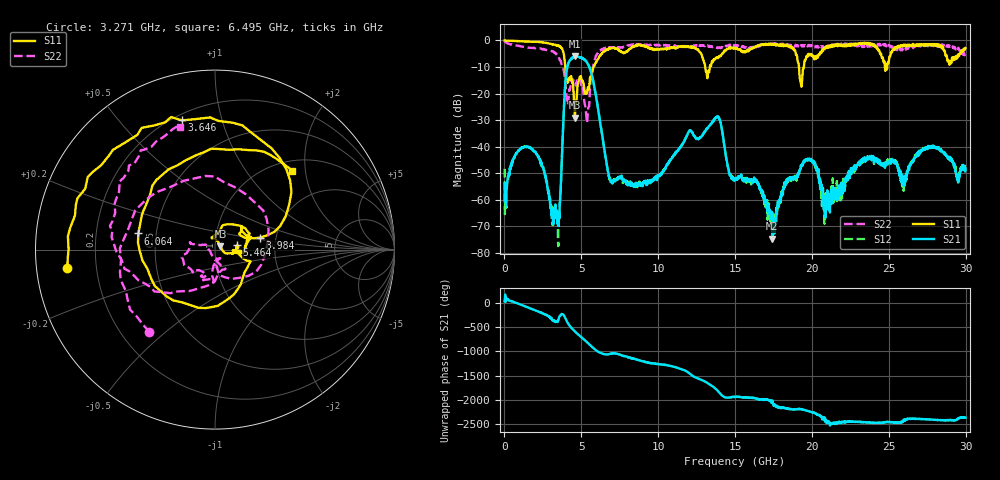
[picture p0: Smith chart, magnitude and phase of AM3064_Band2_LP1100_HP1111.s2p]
# Hz S DB R 50.0
!freq dBS11 angS11 dBS21 angS21 dBS12 angS12 dBS22 angS22
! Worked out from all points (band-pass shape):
!   1600 points, 10 MHz to 29.98 GHz, reference 50 ohm
!   highest |S21| = -6.01 dB at 4.602 GHz (marker M1); lowest = -74.6 dB at 17.42 GHz (marker M2)
!   |S21| within 3 dB of the highest: 4.138 GHz to 5.434 GHz (1.296 GHz wide, 27.1 % of centre)
!   lowest |S11| = -29.0 dB at 4.583 GHz (marker M3), VSWR 1.07, Z = 53.1 + j1.96 ohm
!   |S11| at or under -10 dB: 3.958 GHz to 5.791 GHz (1.834 GHz wide, 37.6 % of centre); 13.06 GHz to 13.35 GHz (297.2 MHz wide, 2.25 % of centre); 19.16 GHz to 19.47 GHz (316.6 MHz wide, 1.64 % of centre)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
!   |S22| runs from -31.0 to -0.3 dB; largest |S21 - S12| = 0.0099
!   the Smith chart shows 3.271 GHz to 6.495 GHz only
!   S11 on the Smith chart (normalised r, x): 3.271 GHz: 0.09, -0.06; 3.646 GHz: 0.23, +0.75; 3.984 GHz: 1.64, +0.23; 5.464 GHz: 1.28, +0.06; 6.064 GHz: 0.40, +0.09; 6.495 GHz: 1.20, +1.70
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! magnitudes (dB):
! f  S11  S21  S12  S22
! 10 MHz  0.0  -53.8  -48.3  -0.3
! 1.659 GHz  -0.5  -40.4  -40.3  -2.7
! 3.271 GHz  -1.6  -64.5  -63.3  -4.6
! 3.646 GHz  -2.6  -56.9  -56.9  -7.7
! 3.984 GHz  -11.8  -14.4  -14.4  -17.5
! 4.583 GHz  -29.0  -6.2  -6.1  -15.5
! 4.602 GHz  -26.2  -6.0  -6.0  -15.8
! 5.015 GHz  -14.6  -6.7  -6.6  -17.2
! 5.464 GHz  -18.0  -9.3  -9.3  -25.2
! 6.064 GHz  -7.2  -24.8  -24.8  -4.7
! 6.495 GHz  -4.2  -40.8  -41.2  -2.9
! 6.983 GHz  -2.9  -52.9  -53.4  -2.5
! 10 GHz  -3.4  -51.1  -50.7  -1.8
! 13.82 GHz  -6.4  -28.7  -28.7  -2.6
! 15 GHz  -2.8  -52.0  -52.1  -1.9
! 16.39 GHz  -2.2  -53.2  -53.3  -2.4
! 17.42 GHz  -1.7  -74.6  -67.4  -1.4
! 19.32 GHz  -17.4  -46.9  -47.0  -1.8
! 19.99 GHz  -5.4  -45.2  -45.5  -1.9
! 20.91 GHz  -2.5  -62.5  -58.0  -2.5
! 25 GHz  -8.2  -45.8  -46.0  -1.7
! 29.98 GHz  -2.8  -48.2  -47.9  -4.7
